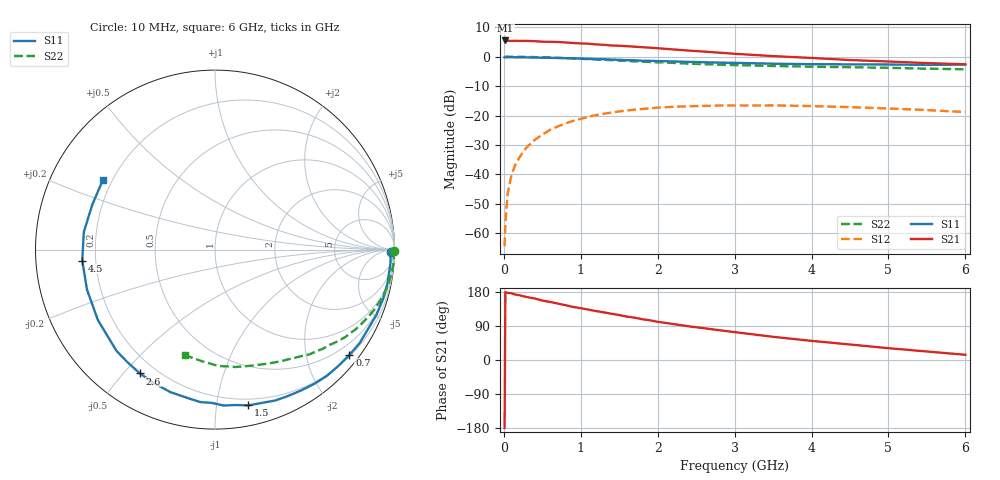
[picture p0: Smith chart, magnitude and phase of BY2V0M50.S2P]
! SIEMENS Small Signal Semiconductors
! BFY420
! Si NPN RF SIEGET Grounded Emitter Transistor in MICRO-X
! VCE = 2 V  IC = 0.5 mA
! Common Emitter S-Parameters:  October  1996
# GHz  S  MA  R  50
!  f  S11  S21  S12  S22
! GHz  MAG  ANG  MAG  ANG  MAG  ANG  MAG  ANG
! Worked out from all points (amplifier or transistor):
!   36 points, 10 MHz to 6 GHz, reference 50 ohm
!   highest |S21| = 5.5 dB at 20 MHz (marker M1)
!   |S21| within 3 dB of that: start of sweep to 2.176 GHz
!   unconditionally stable (mu >= 1): 4.728 GHz to end of sweep
!   at 250 MHz: K = 0.03, MSG = 18.9 dB, |S12| = -32.4 dB
!   at 1.4 GHz: K = 0.19, MSG = 11.4 dB, |S12| = -19.0 dB
!   at 6 GHz: K = 1.42, MAG = 4.3 dB, |S12| = -18.8 dB
!   S11 on the Smith chart (normalised r, x): 10 MHz: 70, -39; 700 MHz: 0.23, -2.88; 1.5 GHz: 0.15, -1.23; 2.6 GHz: 0.14, -0.56; 4.5 GHz: 0.15, -0.04; 6 GHz: 0.16, +0.28
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0.01  0.9784 -0.7  1.89 -179.2  0.0006 87.0  0.9995 -0.3
0.02  0.9744 -1.2  1.892 178.8  0.0015 79.2  0.9989 -0.6
0.05  0.9799 -3.0  1.868 177.2  0.0047 91.0  0.9994 -1.3
0.1  0.9802 -5.5  1.859 176.0  0.0099 87.2  0.9972 -2.7
0.15  0.9779 -8.2  1.865 172.6  0.0146 84.1  0.998 -4.0
0.25  0.9766 -13.7  1.86 168.5  0.0241 81.0  0.994 -6.6
0.4  0.9703 -22.0  1.837 162.4  0.0384 76.1  0.9857 -10.7
0.5  0.9605 -27.5  1.804 156.9  0.0473 72.9  0.978 -13.2
0.7  0.9514 -38.1  1.783 149.0  0.0652 65.9  0.9592 -18.2
0.9  0.9399 -48.6  1.711 140.1  0.0811 59.1  0.9356 -23.0
1.1  0.9194 -58.7  1.666 132.9  0.0951 53.1  0.9115 -27.6
1.5  0.8873 -77.9  1.539 118.6  0.1174 40.9  0.8617 -35.6
1.8  0.8541 -91.2  1.451 107.6  0.1293 33.4  0.8242 -41.0
2.2  0.8322 -107.3  1.332 95.0  0.1408 23.9  0.7861 -47.9
2.6  0.8067 -121.2  1.225 83.9  0.1458 16.2  0.7482 -53.8
3  0.7871 -134.2  1.123 73.6  0.1481 9.3  0.7214 -59.7
3.5  0.7616 -148.9  1.026 61.2  0.1487 2.0  0.6962 -66.2
4  0.7473 -162.6  0.953 50.5  0.1447 -4.1  0.6766 -73.1
4.5  0.7421 -175.3  0.879 40.9  0.139 -9.5  0.6638 -80.2
5  0.7375 172.4  0.83 31.2  0.1316 -13.2  0.6482 -88.4
5.5  0.728 159.9  0.78 22.4  0.1239 -15.8  0.6268 -96.5
6  0.735 148.4  0.744 13.8  0.1145 -16.7  0.6117 -105.6
